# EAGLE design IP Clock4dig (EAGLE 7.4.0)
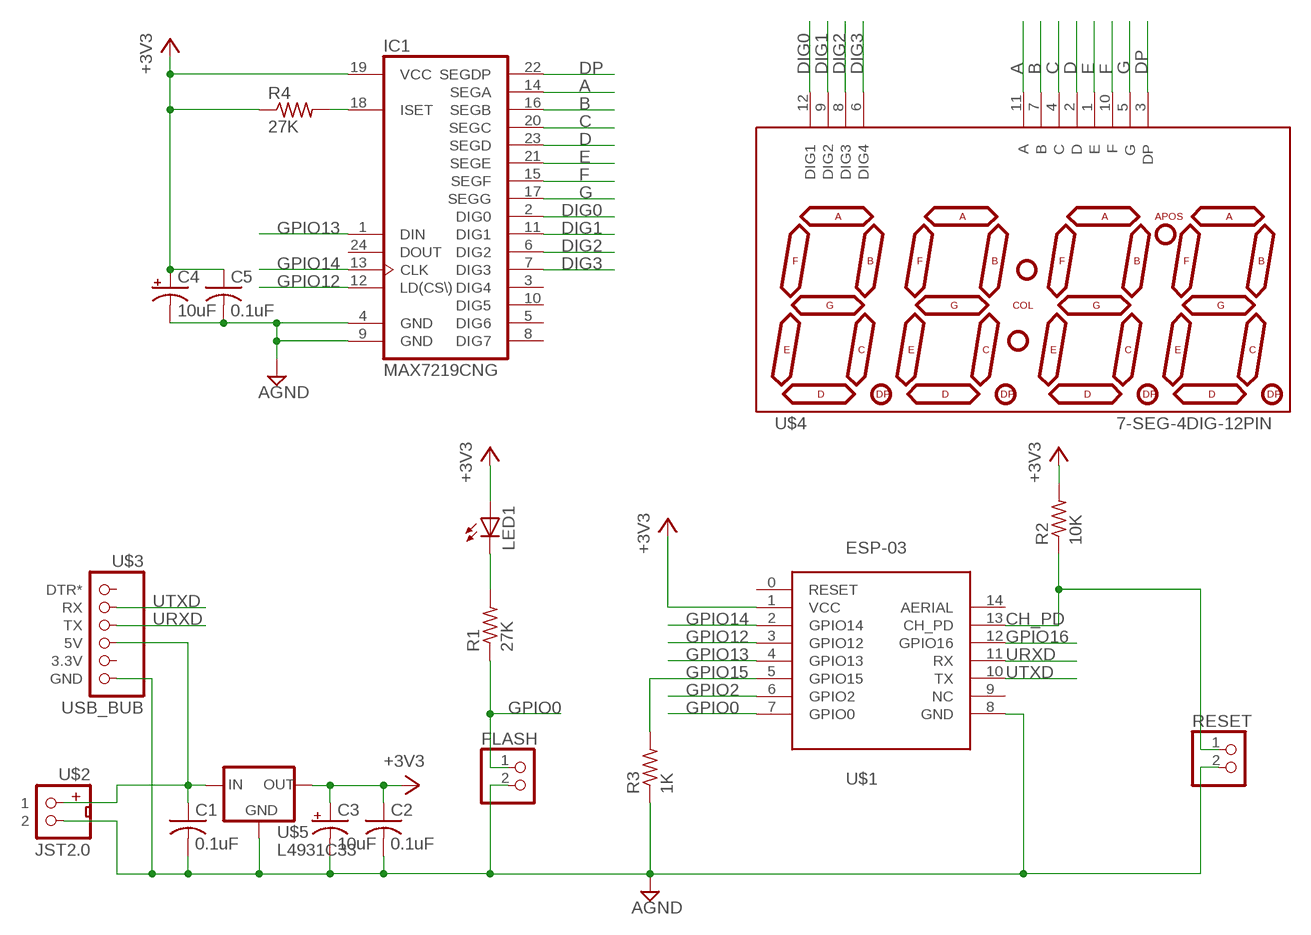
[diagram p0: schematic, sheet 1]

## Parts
C1  0.1uF  C-US050-024X044  [C050-024X044]
C2  0.1uF  C-US025-024X044  [C025-024X044]
C3  10uF  CPOL-USE5-5  [E5-5]
C4  10uF  CPOL-USE5-5  [E5-5]
C5  0.1uF  C-US050-025X075  [C050-025X075]
FLASH  PINHD-1X2  [1X02]
IC1  MAX7219CNG  [DIL24-3]
LED1  LED3MM  [LED3MM]
R1  27K  R-US_0204/7  [0204/7]
R2  10K  R-US_0204/7  [0204/7]
R3  1K  R-US_0204/7  [0204/7]
R4  27K  R-US_0204/2V  [0204V]
RESET  PINHD-1X2  [1X02]
U$1  ESP-03  [ESP-03]
U$2  JST2.0  [JST2.0]
U$3  USB_BUB  [USB_BUB]
U$4  7-SEG-4DIG-12PIN  [7-SEG-4DIG-12PIN]
U$5  L4931C33  [TO92-INLINE]

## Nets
5V: C1.1 U$2.1 U$3.5V U$5.3(IN)
+3V3: C2.1 C3.+ C4.+ C5.1 IC1.19(VCC) LED1.A R2.2 R4.1 U$1.1(VCC) U$5.1(OUT)
A: IC1.14(SEGA) U$4.11(A)
AGND: C1.2 C2.2 C3.- C4.- C5.2 FLASH.2 IC1.4(GND) IC1.9(GND) R3.1 RESET.2 U$1.8(GND) U$2.2 U$3.GND U$5.2(GND)
B: IC1.16(SEGB) U$4.7(B)
C: IC1.20(SEGC) U$4.4(C)
CH_PD: R2.1 RESET.1 U$1.13(CH_PD)
D: IC1.23(SEGD) U$4.2(D)
DIG0: IC1.2(DIG0) U$4.12(DIG1)
DIG1: IC1.11(DIG1) U$4.9(DIG2)
DIG2: IC1.6(DIG2) U$4.8(DIG3)
DIG3: IC1.7(DIG3) U$4.6(DIG4)
DP: IC1.22(SEGDP) U$4.3(DP)
E: IC1.21(SEGE) U$4.1(E)
F: IC1.15(SEGF) U$4.10(F)
G: IC1.17(SEGG) U$4.5(G)
GPIO0: FLASH.1 R1.1 U$1.7(GPIO0)
GPIO2: U$1.6(GPIO2)
GPIO12: IC1.12(LD(CS\)) U$1.3(GPIO12)
GPIO13: IC1.1(DIN) U$1.4(GPIO13)
GPIO14: IC1.13(CLK) U$1.2(GPIO14)
GPIO15: R3.2 U$1.5(GPIO15)
GPIO16: U$1.12(GPIO16)
N$1: IC1.18(ISET) R4.2
N$5: LED1.K(C) R1.2
URXD: U$1.11(RX) U$3.TX
UTXD: U$1.10(TX) U$3.RX
Unconnected: IC1.3(DIG4) IC1.5(DIG6) IC1.8(DIG7) IC1.10(DIG5) IC1.24(DOUT) U$1.0(RESET) U$1.9(NC) U$1.14(AERIAL) U$3.3.3V U$3.DTR*

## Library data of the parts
C1 C2 C5 = rcl:C-US: CAPACITOR, American symbol
C3 C4 = rcl:CPOL-US: POLARIZED CAPACITOR, American symbol
FLASH RESET = pinhead:PINHD-1X2: PIN HEADER
IC1 = MTS_Custom:MAX7219CNG: LED DISPLAY DRIVER; MF: MAXIM; MPN: MAX7219CNG; OC_FARNELL: 1523914; OC_NEWARK: 34C4018
LED1 = adafruit:LED: LED
R1-R4 = rcl:R-US_: RESISTOR, American symbol
U$1 = Temp1:ESP-03
U$2 = MTS_Custom:JST2.0: JST 2.0 2 pin connector 2mm spacing
U$3 = MTS_Custom:USB_BUB
U$4 = MTS_Custom:7-SEG-4DIG-12PIN
U$5 = MTS_Custom:L4931C33: Voltage Regulator 3.3Vdc LDO (0.4V) 250mA output

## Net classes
0 default: width 0.4 mm, clearance 0.3 mm
1 power: width 0.6 mm, clearance 0.3 mm

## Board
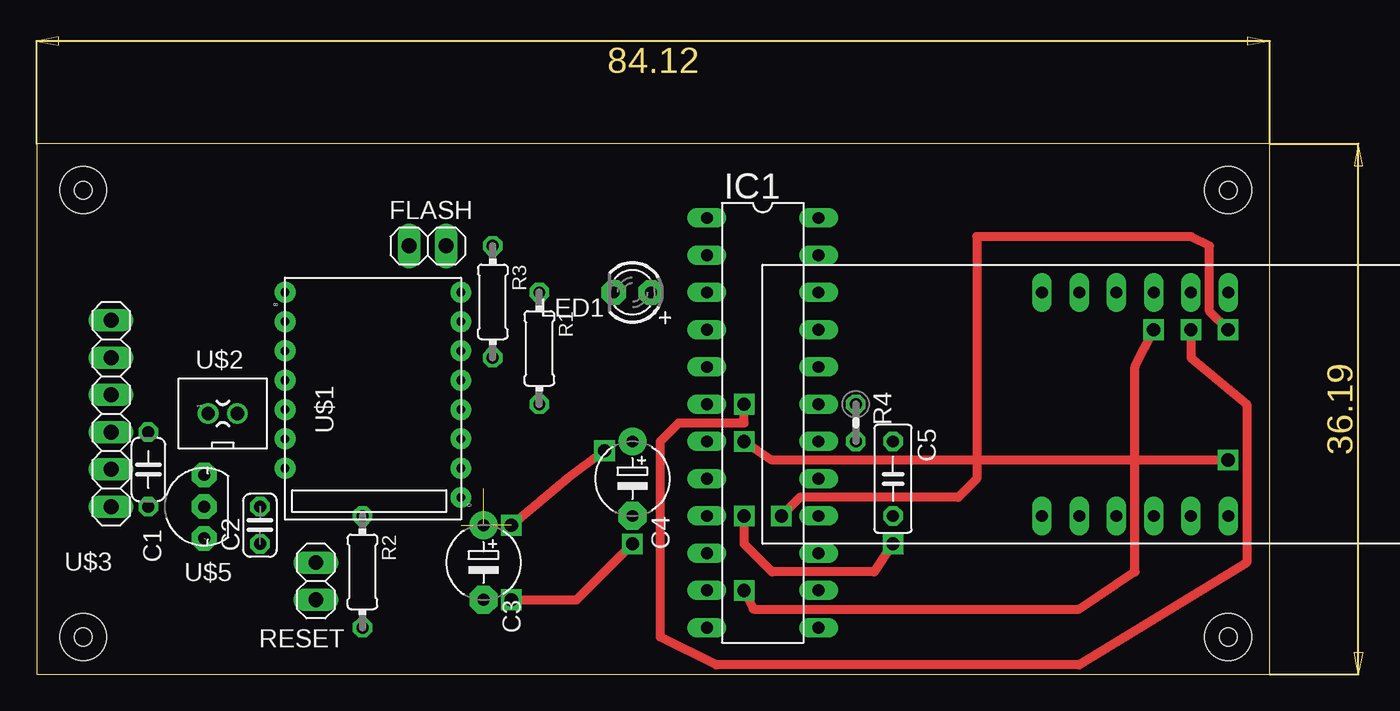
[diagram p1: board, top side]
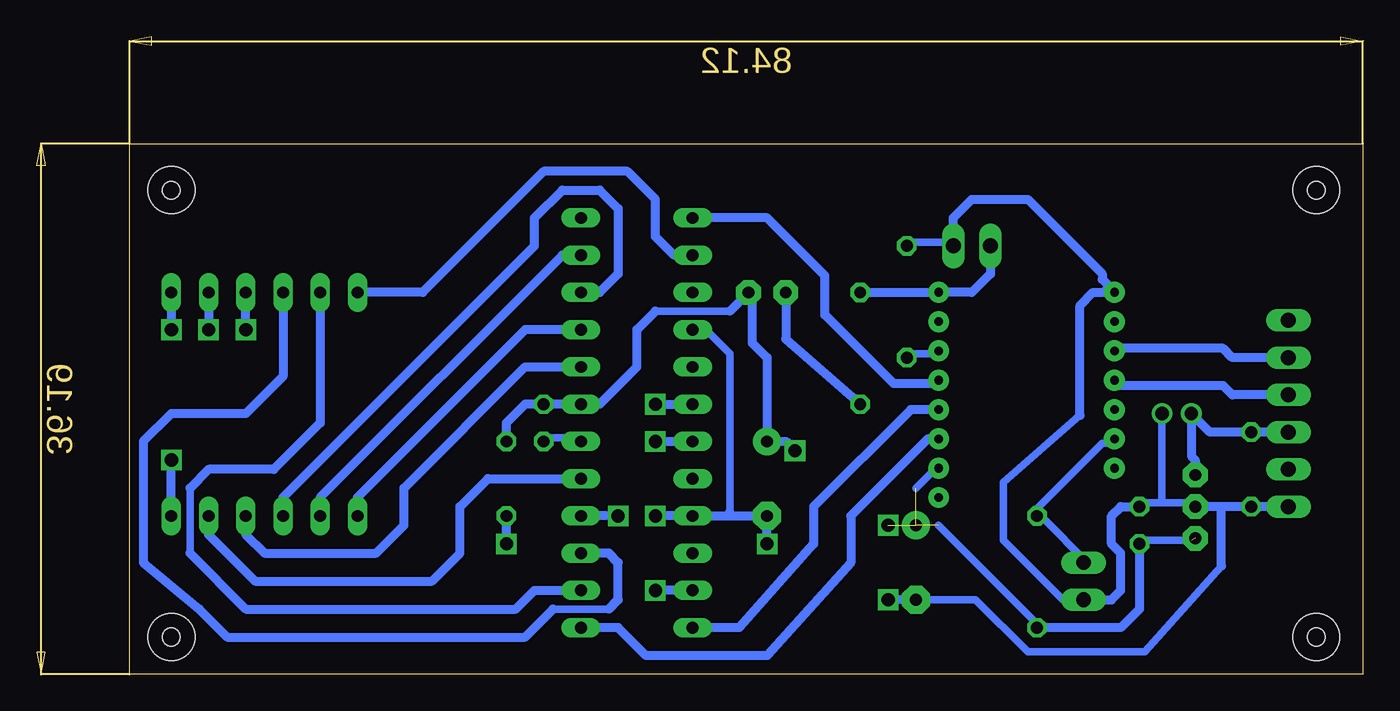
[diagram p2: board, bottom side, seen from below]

Size 90.47 x 43.48 mm. Coordinates in mm from the lower left corner, seen from the top.
Outline: 0,0 84.12,0 84.12,36.19 0,36.19 0,0
Copper layers (1*16): Top 0.035mm / dielectric 1.5mm / Bottom 0.035mm
Design rules "NewMTS": minimum track width 20mil, minimum drill 24mil, track to track 20mil, track to pad 20mil, pad to pad 8mil, via to via 8mil, smd to smd 8mil, copper to edge 40mil, drill to drill 8mil, minimum pad ring 10mil, minimum via ring 10mil, stop-mask expansion 4mil, vias tented up to drill 0mil, thermal gap 10mil
Holes 3.2 mm at 81.28,2.54 3.17,2.54 3.17,33.02 81.28,33.02
Holes 1.2 mm at 3.17,33.02 3.17,2.54 81.28,2.54 81.28,33.02

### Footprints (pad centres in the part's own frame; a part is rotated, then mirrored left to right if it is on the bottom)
C050-024X044 = drill 0.813 octagon: 1 -2.54,0; 2 2.54,0
C025-024X044 = drill 0.813 octagon: 1 -1.27,0; 2 1.27,0
E5-5 = drill 0.813 pad 1.905: + -2.54,0 | drill 0.813 pad 1.905 octagon: - 2.54,0
C050-025X075 = drill 0.813 octagon: 1 -2.54,0; 2 2.54,0
1X02 = drill 1.016 long: 1 -1.27,0; 2 1.27,0
DIL24-3 = drill 0.813 long: 1 -13.97,-3.81; 2 -11.43,-3.81; 3 -8.89,-3.81; 4 -6.35,-3.81; 5 -3.81,-3.81; 6 -1.27,-3.81; 7 1.27,-3.81; 8 3.81,-3.81; 9 6.35,-3.81; 10 8.89,-3.81; 11 11.43,-3.81; 12 13.97,-3.81; 13 13.97,3.81; 14 11.43,3.81; 15 8.89,3.81; 16 6.35,3.81; 17 3.81,3.81; 18 1.27,3.81; 19 -1.27,3.81; 20 -3.81,3.81; 21 -6.35,3.81; 22 -8.89,3.81; 23 -11.43,3.81; 24 -13.97,3.81
LED3MM = drill 0.813 pad 1.676 octagon: A -1.27,0; K 1.27,0
0204/7 = drill 0.813 octagon: 1 -3.81,0; 2 3.81,0
0204V = drill 0.813 octagon: 1 -1.27,0; 2 1.27,0
ESP-03 = drill 0.6 pad 1.422: 0 -7,-1; 1 -5,-1; 2 -3,-1; 3 -1,-1; 4 1,-1; 5 3,-1; 6 5,-1; 7 7,-1; 8 7,11; 9 5,11; 10 3,11; 11 1,11; 12 -1,11; 13 -3,11; 14 -5,11
JST2.0 = drill 0.9 pad 1.016: 1 0,-1; 2 0,1
USB_BUB = drill 1.016 long: 3.3V -3.81,0; 5V -1.27,0; DTR* 6.35,0; GND -6.35,0; RX 3.81,0; TX 1.27,0
7-SEG-4DIG-12PIN = drill 0.813 long: 1 -6.35,-7.62; 2 -3.81,-7.62; 3 -1.27,-7.62; 4 1.27,-7.62; 5 3.81,-7.62; 6 6.35,-7.62; 7 6.35,7.62; 8 3.81,7.62; 9 1.27,7.62; 10 -1.27,7.62; 11 -3.81,7.62; 12 -6.35,7.62
TO92-INLINE = drill 0.813 pad 1.676 octagon: 1 -2.159,0; 2 0,0; 3 2.159,0

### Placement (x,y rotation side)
C1  7.62,13.97 270 top
C2  15.24,10.16 90 top
C3  30.48,7.62 270 top
C4  40.64,13.34 270 top
C5  58.42,13.34 270 top
FLASH  26.67,29.21 0 top
IC1  49.53,17.14 270 top
LED1  40.64,26.04 180 top
R1  34.29,22.23 270 top
R2  22.23,6.99 270 top
R3  31.11,25.4 270 top
R4  55.88,17.14 270 top
RESET  19.05,6.35 270 top
U$1  27.94,19.05 90 top
U$2  12.7,17.78 270 top
U$3  5.08,17.78 90 top
U$4  74.93,18.41 0 top
U$5  11.43,11.43 90 top

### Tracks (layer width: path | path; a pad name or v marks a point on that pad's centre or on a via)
5V
  Bottom 0.61: U$3.5V C1.1 10.43,16.51 U$2.1 11.7,14.88 11.43,14.61 U$5.3
+3V3  (via drill 0.9)  (4 unrouted)
  Top 0.61: v38.73,15.24 36.2,13.34 v32.38,10.16
  Bottom 0.508: 30.48,12.7 29.46,13.72 28.96,13.72 U$1.1 | 11.68,9.14 15.24,9.14 C2.1 | 28.96,10.16 22.35,3.56 R2.2 | 41.66,25.78 LED1.A | 58.42,16.13 C5.1 | 48.26,24.77 43.18,24.77
  Bottom 0.61: 48.26,24.77 49.53,23.5 49.53,20.95 52.07,18.41 IC1.19 R4.1 57.15,18.41 58.42,17.14 58.42,16.13 | 43.18,24.77 LED1.A | C2.1 15.24,4.45 16.51,3.17 R2.2 | 41.66,25.78 41.66,22.61 40.64,21.59 C4.+ 39.37,15.88 v38.73,15.24
A
  Bottom 0.508: 80.01,12.7 80.01,8.26
  Bottom 0.61: U$4.11 71.12,17.14 74.3,13.97 78.74,13.97 80.01,12.7 | 80.01,8.26 76.2,4.45 57.78,4.45 56.52,5.71 IC1.14
AGND  (via drill 0.9)
  Top 0.61: v48.26,10.79 48.26,8.89 50.16,6.99 57.15,6.99 v58.42,8.89 | v32.38,5.08 36.83,5.08 v40.64,8.89
  Bottom 0.508: 43.18,11.05 43.18,21.84 44.58,23.24 45.72,23.24 IC1.4 | R3.1 30.99,29.46 27.94,29.46 FLASH.2 | 13.72,11.68 11.68,11.68 U$5.2 | 13.72,11.68 15.24,11.68 C2.2 | 13.72,11.68 13.72,17.78 U$2.2 | C3.- 26.42,5.08 22.86,1.52 14.86,1.52 9.65,7.37 | 19.3,17.65 24.51,13.08 24.51,9.14 20.45,5.08 RESET.2
  Bottom 0.61: v48.26,10.79 IC1.9 43.18,10.79 | v58.42,8.89 C5.2 | RESET.2 17.14,5.08 16.51,5.71 16.51,8.26 17.14,8.89 17.14,10.79 16.51,11.43 C2.2 | 43.18,10.79 C4.- v40.64,8.89 | 43.18,11.05 43.18,10.79 | C3.- v32.38,5.08 | 27.94,29.46 27.94,31.11 26.67,32.38 22.86,32.38 17.78,27.3 17.78,26.92 17.27,26.42 | 19.3,17.65 19.3,25.15 18.41,26.04 17.65,26.04 17.27,26.42 | U$3.GND C1.2 9.53,11.43 | 9.53,11.43 U$5.2 | 9.65,7.37 9.65,11.3 9.53,11.43 | 17.27,26.42 17.27,26.38 U$1.8
B  (via drill 0.9)
  Top 0.61: v81.28,23.5 80.01,24.77 80.01,29.21 78.74,29.84 64.14,29.84 64.14,13.34 62.87,12.06 52.07,12.06 v50.8,10.79
  Bottom 0.61: U$4.7 v81.28,23.5 | v50.8,10.79 IC1.16
C
  Bottom 0.61: U$4.4 76.2,9.53 74.93,8.26 67.31,8.26 65.41,10.16 65.41,12.7 57.15,20.95 IC1.20
CH_PD
  Bottom 0.508: RESET.1 18.8,7.62 21.84,10.67 R2.1 22.35,11.18 17.78,15.75 17.27,15.75 U$1.13
D
  Bottom 0.61: U$4.2 71.12,12.06 54.61,28.57 IC1.23
DIG0
  Bottom 0.61: IC1.2 46.99,28.57 48.26,29.84 48.26,32.38 50.16,34.29 55.88,34.29 64.14,26.04 U$4.12
DIG1  (via drill 0.9)
  Top 0.61: v48.26,5.71 48.9,4.45 71.12,4.45 74.93,6.99 74.93,20.95 v76.2,23.5
  Bottom 0.61: IC1.11 v48.26,5.71 | v76.2,23.5 U$4.9
DIG2  (via drill 0.9)
  Top 0.61: v78.74,23.5 78.74,21.59 82.55,18.41 82.55,7.62 71.12,0.64 46.35,0.64 42.55,2.54 42.55,15.88 43.81,17.14 48.26,17.14 v48.26,18.41
  Bottom 0.61: U$4.8 v78.74,23.5 | v48.26,18.41 IC1.6
DIG3  (via drill 0.9)
  Top 0.61: v81.28,14.61 50.16,14.61 v48.26,15.88
  Bottom 0.61: U$4.6 v81.28,14.61 | v48.26,15.88 IC1.7
DP
  Bottom 0.61: U$4.3 73.66,12.06 56.52,29.21 56.52,31.11 54.61,33.02 52.07,33.02 50.8,31.75 50.8,27.3 52.07,26.04 IC1.22
E
  Bottom 0.61: IC1.21 57.15,23.5 68.58,12.06 U$4.1
F
  Bottom 0.508: 55.24,4.45 51.44,4.45
  Bottom 0.61: U$4.10 73.66,20.32 76.2,17.78 81.28,17.78 83.19,15.88 83.19,7.62 79.38,4.45 77.47,2.54 57.15,2.54 55.24,4.45 | 51.44,4.45 50.8,5.08 50.8,7.62 51.44,8.26 IC1.15
G
  Bottom 0.61: U$4.5 78.74,9.53 75.56,6.35 63.5,6.35 61.59,8.26 61.59,11.43 59.69,13.34 IC1.17
GPIO0
  Bottom 0.61: R1.1 28.95,26.04 U$1.7 28.93,26.04 26.67,26.04 25.4,27.3 FLASH.1
GPIO12
  Bottom 0.61: U$1.3 30.84,18.05 37.47,11.43 37.47,8.89 42.55,3.17 IC1.12
GPIO13
  Bottom 0.508: 28.96,19.81 U$1.4
  Bottom 0.61: 28.96,19.81 32,19.81 36.7,24.51 36.7,27.18 40.64,31.11 IC1.1
GPIO14
  Bottom 0.61: U$1.2 29.67,16.05 34.92,10.79 34.92,7.62 40.64,1.27 48.9,1.27 50.8,3.17 IC1.13
GPIO15
  Bottom 0.508: R3.2 30.99,21.84 28.96,21.84 U$1.5
N$1
  Bottom 0.508: IC1.18 53.34,16.13 55.88,16.13 R4.2
N$5
  Bottom 0.61: LED1.K 39.37,22.86 R1.2
URXD
  Bottom 0.61: U$3.TX 8.89,19.05 9.53,19.68 16.57,19.68 U$1.11
UTXD
  Bottom 0.61: U$3.RX 8.89,21.59 9.53,22.23 16.77,22.23 U$1.10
